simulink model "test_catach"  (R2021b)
settings: Solver=FixedStepAuto  StartTime=0.0  StopTime=inf  FixedStep=0.1  RelTol=1e-3

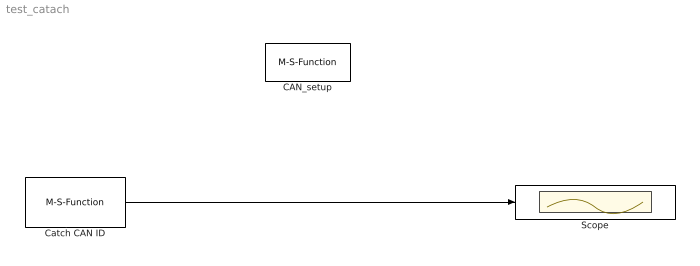
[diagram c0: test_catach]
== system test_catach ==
  CAN_setup : M-S-Function  Priority=1  FunctionName=CAN_setup2  Parameters=g1_cmbPortName, g2_cmbBaudRate,g3_chkEcho,g59_chkTerminator,g4_cmbObjectID,g5_chkEnableSync,g6_rdoSyncSource,g7_ediSyncCANID,g8_chkSyncExtended,g9_ediSyncPeriod,g10_chkRxWDEnable,g11_cmbRxWDDLC,g55_chkRxWDCANID,g56_chkRxWDExtended,g12_cmbRxWDLen,g13_cmbRxWDStartPos,g14_ediRxWDPeriod,g_60_cmbRxWDMode,g15_chkTxWDEnable,g16_cmbTxWDDLC,g57_chkTxWDCANID,g58_chkTxWDExtended,g17_cmbTxWDLen,g18_cmbTxWDSta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  mask(CAN Bus controller setup){g1_cmbPortName="COM17", g2_cmbBaudRate=250000, g3_chkEcho=off, g59_chkTerminator=on, g4_cmbObjectID=0, g5_chkEnableSync=off, g6_rdoSyncSource=Sync by dedicated Receiving frame, g7_ediSyncCANID=123, g8_chkSyncExtended=off, g9_ediSyncPeriod=500, g10_chkRxWDEnable=off, g11_cmbRxWDDLC=1, g55_chkRxWDCANID=234, g56_chkRxWDExtended=off, g12_cmbRxWDLen=1, g13_cmbRxWDStartPos=1, g14_ediRxWDPeriod=500, g_60_cmbRxWDMode=0, g15_chkTxWDEnable=off, g16_cmbTxWDDLC=1, g57_chkTxWDCANID=345, g58_chkTxWDExtended=off, g17_cmbTxWDLen=1, g18_cmbTxWDStartPos=1, g19_ediTxWDPeriod=500, g_61_cmbTxWDMode=0, g20_ediF1=0, g21_chkExt4F1=off, g22_ediF2=0, g23_chkExt4F2=off, g24_ediF3=0, g25_chkExt4F3=off, g26_ediF4=0, g27_chkExt4F4=off, g28_ediF5=0, g29_chkExt4F5=off, g30_ediF6=0, g31_chkExt4F6=off, g32_ediF7=0, g33_chkExt4F7=off, g34_ediF8=0, g35_chkExt4F8=off, g36_ediM1=0, g37_ediF9=0, g38_chkExt4F9=off, g39_ediF10=0, g40_chkExt4F10=on, g41_ediF11=0, g42_chkExt4F11=on, g43_ediF12=0, g44_chkExt4F12=on, g45_ediM2=0, g46_ediF13=0, g47_chkExt4F13=on, g48_ediF14=0, g49_chkExt4F14=on, g50_ediF15=0, g51_chkExt4F15=on, g52_ediF16=0, g53_chkExt4F16=on, g54_ediM3=0}
      mask prompts: g1_cmbPortName "Connect to:"; g2_cmbBaudRate "CAN Bus Baud Rate:"; g3_chkEcho "Echo On"; g59_chkTerminator "Enable 120 Ω terminator"; g4_cmbObjectID "Object ID for multiple CAN bus controllers:"; g5_chkEnableSync "Enable Sync:"; g6_rdoSyncSource "Sync Source Selection"; g7_ediSyncCANID "SyncCAN ID:"; g8_chkSyncExtended "Sync uses extended CAN ID"; g9_ediSyncPeriod "Sync periods in ms:"; g10_chkRxWDEnable "Rx Watchdog Enable"; g11_cmbRxWDDLC "Rx Watchdog Frame DLC"; g55_chkRxWDCANID "RxWatchdogCAN ID:"; g56_chkRxWDExtended "RxWatchdog uses extended ID"; g12_cmbRxWDLen "RxWatchdog Counter byte qty"; g13_cmbRxWDStartPos "RxWatchdog Start position:"; g14_ediRxWDPeriod "RxWatchdog Periods:"; g_60_cmbRxWDMode "RxWatchdog Mode"; g15_chkTxWDEnable "TxWatchdog Enable"; g16_cmbTxWDDLC "Tx Watchdog Frame DLC"; g57_chkTxWDCANID "TxWatchdogCAN ID:"; g58_chkTxWDExtended "TxWatchdog uses extended ID"; g17_cmbTxWDLen "TxWatchdog Counter byte qty"; g18_cmbTxWDStartPos "TxWatchdog Start position:"; g19_ediTxWDPeriod "TxWatchdog Periods:"; g_61_cmbTxWDMode "TxWatchdog Mode"; g20_ediF1 "Filter1"; g21_chkExt4F1 "Extended"; g22_ediF2 "Filter2"; g23_chkExt4F2 "Extended"; g24_ediF3 "Filter3"; g25_chkExt4F3 "Extended"; g26_ediF4 "Filter4"; g27_chkExt4F4 "Extended"; g28_ediF5 "Filter5"; g29_chkExt4F5 "Extended"; g30_ediF6 "Filter6"; g31_chkExt4F6 "Extended"; g32_ediF7 "Filter7"; g33_chkExt4F7 "Extended"; g34_ediF8 "Filter8"; g35_chkExt4F8 "Extended"; g36_ediM1 "Mask1"; g37_ediF9 "Filter9"; g38_chkExt4F9 "Extended"; g39_ediF10 "Filter10"; g40_chkExt4F10 "Extended"; g41_ediF11 "Filter11"; g42_chkExt4F11 "Extended"; g43_ediF12 "Filter12"; g44_chkExt4F12 "Extended"; g45_ediM2 "Mask2"; g46_ediF13 "Filter13"; g47_chkExt4F13 "Extended"; g48_ediF14 "Filter14"; g49_chkExt4F14 "Extended"; g50_ediF15 "Filter15"; g51_chkExt4F15 "Extended"; g52_ediF16 "Filter16"; g53_chkExt4F16 "Extended"; g54_ediM3 "Mask3"
      mask help: It sets up CAN Bus controller.. You must firstly set up CAN Bus controller before you use any CAN bus controller block. Parameter "Object ID for multilple CAN bus controllers" is for CAN bus controller object ID. We could use multiple CAN bus controllers, so we use this parameter to identify different CAN bus controller objects for other CAN Bus controller operation blocks.
  Catch CAN ID : M-S-Function  FunctionName=catchCANID2  Parameters="g1_ObjectID, g2_CANID,  g3_Extended"  mask{g1_ObjectID=0, g2_CANID=123, g3_Extended=on}
      mask prompts: g1_ObjectID "Object ID for multiple CAN bus controllers:"; g2_CANID "Catch CAN ID:"; g3_Extended "Extended"
  Scope : Scope
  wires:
  Catch CAN ID/1 -> Scope/1
